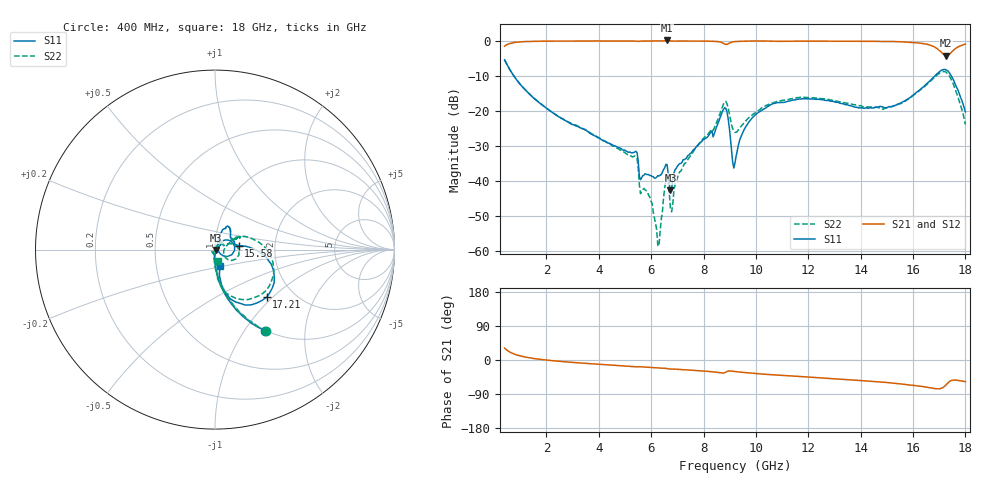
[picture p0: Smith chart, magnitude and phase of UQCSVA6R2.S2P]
!  Part Number  UQCSVA6R2  Mounting Orientation: Horizontal
!  Description: Ultra Low ESR Microwave capacitors
!  Application: Coupling, Bypass, Tuning, DC Block
!  Filters, Matching
# GHZ S DB R 50
! Freq  |S11|  S11 Ph  |S21|  S21 Ph  |S12|  S12 Ph  |S22|  S22 Ph
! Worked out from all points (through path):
!   401 points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, 400 MHz to 18 GHz, reference 50 ohm
!   highest |S21| = 0.08 dB at 6.604 GHz (marker M1); lowest = -4.2 dB at 17.25 GHz (marker M2)
!   group delay of S21, straight-line fit = 12.6 ps
!   lowest |S11| = -42.7 dB at 6.736 GHz (marker M3), VSWR 1.01, Z = 50.7 - j0.144 ohm
!   |S11| at or under -10 dB: 749.2 MHz to 16.84 GHz (16.09 GHz wide, 183 % of centre); 17.46 GHz to end of sweep
!   |S22| runs from -58.5 to -5.4 dB; largest |S21 - S12| = 0.008
!   S11 on the Smith chart (normalised r, x): 400 MHz: 0.99, -1.25; 15.58 GHz: 1.30, +0.06; 17.21 GHz: 1.47, -0.92; 18 GHz: 1.04, -0.19
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0.4  -5.46 -58.2  -1.56 31.3  -1.57 31.3  -5.43 -57.6
1.588  -16.84 -85.1  -0.15 3.3  -0.15 3.2  -16.78 -84.8
3.348  -24.99 -92.7  -0.08 -8.1  -0.07 -8.1  -24.95 -93.9
5.372  -31.67 -90.2  -0.10 -17.7  -0.09 -17.7  -32.87 -121.9
5.636  -39.00 -75.7  -0.09 -18.2  -0.08 -18.2  -42.79 -118.0
5.944  -38.41 -56.9  -0.07 -19.7  -0.06 -19.6  -44.53 -121.0
6.296  -38.54 -25.5  -0.07 -21.2  -0.06 -21.1  -58.54 114.7
6.604  -35.26 -34.1  0.08 -22.9  0.08 -22.7  -38.40 29.0
6.736  -42.67 -11.1  -0.05 -23.8  -0.06 -23.8  -48.11 18.3
7.132  -34.98 23.5  -0.08 -25.1  -0.07 -25.0  -37.21 64.9
8.452  -25.46 53.9  -0.18 -32.0  -0.17 -31.8  -24.05 25.0
8.804  -19.10 10.8  -0.92 -33.7  -0.91 -33.6  -17.46 -2.0
9.2  -34.78 41.2  -0.24 -30.5  -0.23 -30.4  -26.11 -12.3
9.508  -26.00 70.1  -0.14 -32.8  -0.12 -32.6  -23.70 16.9
10.036  -20.73 70.3  -0.06 -35.9  -0.05 -35.8  -20.19 26.9
12.148  -16.59 57.7  -0.13 -45.9  -0.12 -45.7  -16.29 25.8
15.096  -18.79 16.1  -0.19 -60.2  -0.18 -60.0  -18.77 32.4
15.58  -17.50 9.5  -0.32 -63.5  -0.30 -63.4  -17.70 31.0
16.636  -11.49 -5.7  -1.21 -73.2  -1.21 -72.9  -11.71 6.8
17.208  -8.16 -42.6  -4.09 -69.2  -4.07 -68.9  -8.79 -39.9
17.252  -8.27 -47.1  -4.23 -66.1  -4.20 -65.7  -8.91 -44.9
18  -20.26 -71.7  -0.95 -57.3  -0.95 -57.1  -23.85 -74.3
